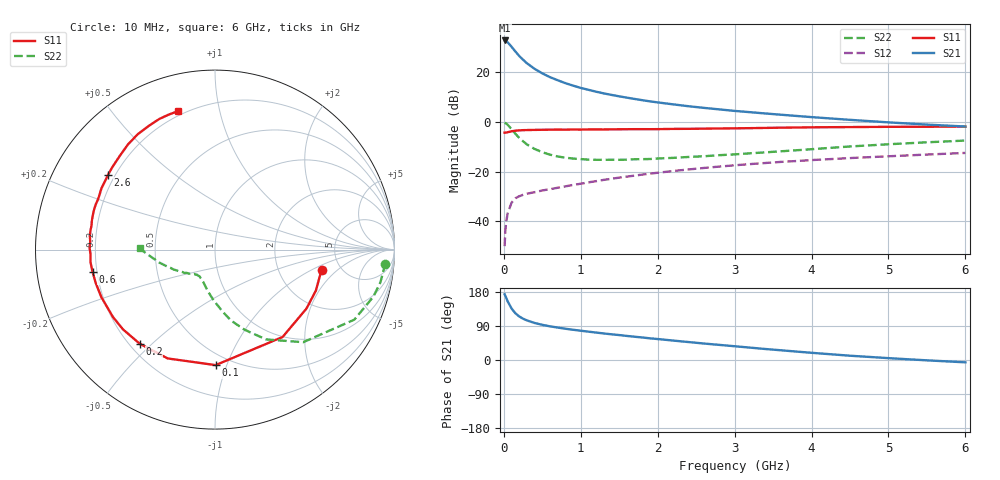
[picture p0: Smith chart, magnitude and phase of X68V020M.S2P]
! SIEMENS Small Signal Semiconductors
! BFP193W
! Si NPN RF Bipolar Junction Transistor in SOT343
! VCE = 8 V  IC = 20 mA
! Common Emitter S-Parameters:  April 1994
# GHz  S  MA  R  50
!  f  S11  S21  S12  S22
! GHz  MAG  ANG  MAG  ANG  MAG  ANG  MAG  ANG
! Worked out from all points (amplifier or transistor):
!   40 points, 10 MHz to 6 GHz, reference 50 ohm
!   highest |S21| = 32.6 dB at 10 MHz (marker M1)
!   |S21| within 3 dB of that: start of sweep to 112.9 MHz
!   unconditionally stable (mu >= 1): 1.01 GHz to 4.56 GHz
!   at 200 MHz: K = 0.33, MSG = 28.1 dB, |S12| = -29.9 dB
!   at 1.5 GHz: K = 1.09, MAG = 14.5 dB, |S12| = -22.4 dB
!   at 6 GHz: K = 0.95, MSG = 5.3 dB, |S12| = -12.5 dB
!   lowest NFmin = 1.40 dB at 450 MHz
!   S11 on the Smith chart (normalised r, x): 10 MHz: 3.57, -1.27; 100 MHz: 0.42, -0.91; 200 MHz: 0.24, -0.46; 600 MHz: 0.18, -0.09; 2.6 GHz: 0.17, +0.31; 6 GHz: 0.18, +0.75
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0.01  0.6041 -10.8  42.67 173.4  0.0032 84.2  0.9521 -4.7
0.02  0.6067 -22.1  42.29 169.1  0.0067 79.7  0.9396 -11.2
0.03  0.6064 -32.8  41.54 164.2  0.0097 76.6  0.9202 -16.6
0.05  0.6156 -52.3  39.15 154.6  0.0146 69.1  0.8689 -26.7
0.1  0.6436 -89.7  31.98 136.1  0.0238 54.1  0.7124 -46.4
0.15  0.6612 -113.5  25.64 123.3  0.0292 45.9  0.5754 -60.4
0.2  0.6716 -128.7  20.85 115.0  0.0321 41.5  0.4745 -69.9
0.25  0.6785 -139.1  17.5 109.0  0.0343 39.5  0.4056 -77.2
0.3  0.6814 -146.5  14.9 104.5  0.0361 38.5  0.3509 -82.7
0.4  0.6865 -157.3  11.5 97.7  0.0387 38.6  0.2846 -91.3
0.5  0.6902 -164.5  9.342 92.8  0.0419 40.4  0.2448 -97.8
0.6  0.6933 -169.8  7.84 88.8  0.0444 41.5  0.2186 -103.1
0.8  0.6938 -177.7  5.944 82.5  0.0506 45.4  0.1903 -110.5
1.1  0.7016 173.8  4.37 74.8  0.0609 48.9  0.174 -118.6
1.3  0.7009 168.9  3.701 70.0  0.0683 50.6  0.1724 -122.1
1.6  0.7085 162.9  3.041 63.5  0.0794 52.0  0.1737 -126.5
2.2  0.7188 151.7  2.233 51.3  0.1028 51.9  0.1886 -134.9
2.6  0.7271 145.0  1.898 43.5  0.1184 50.7  0.2033 -140.3
3.2  0.7443 135.5  1.556 32.7  0.1415 47.9  0.2329 -148.5
4.5  0.7821 118.0  1.092 11.3  0.1869 40.2  0.3193 -167.0
5.5  0.7946 109.3  0.877 -0.9  0.2199 34.4  0.3873 -177.2
6  0.799 104.9  0.802 -6.2  0.2371 31.9  0.4198 178.9
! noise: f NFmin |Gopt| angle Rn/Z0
0.45  1.4  0.3  160  0.1
0.9  1.45  0.34  172  0.11
1.8  2.2  0.56  -148  0.2
